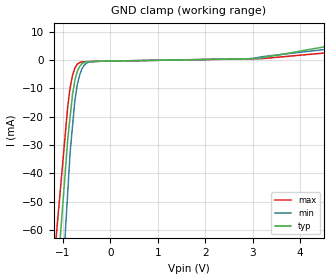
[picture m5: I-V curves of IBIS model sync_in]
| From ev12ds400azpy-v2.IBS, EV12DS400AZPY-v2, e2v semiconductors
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[Model] sync_in
Model_type Input
Vinl = 1.15000V
Vinh = 1.35000V
C_comp 573.000fF 559.000fF 587.000fF
| variable typ   min   max
[Voltage Range] 3.30000V 3.15000V 3.45000V
[POWER Clamp Reference] 3.30000V 3.15000V 3.45000V
[GND Clamp Reference] 0.00000V 0.00000V 0.00000V
[Temperature Range]   25   110   -40
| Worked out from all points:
|   GND clamp passes 1 mA (typ) near -0.57 V on its own axis
[GND Clamp]
-3.3V     -556.2mA   -716.5mA   -469.2mA
-900mV    -27.91mA   -46.58mA   -16.34mA
-850mV    -20.04mA   -32.62mA   -9.785mA
-800mV    -12.18mA   -23.45mA   -5.383mA
-750mV    -7.147mA   -14.29mA   -2.781mA
-700mV    -3.992mA   -8.686mA   -1.463mA
-650mV    -2.306mA   -5.331mA   -888.1uA
-600mV    -1.286mA   -3.039mA   -609.2uA
-550mV    -785.3uA   -1.74mA    -578.7uA
-450mV    -530.2uA   -687uA     -517.8uA
3.15V     668uA      1.043mA    518uA
6.6V      10.84mA    7.725mA    5.659mA
[POWER Clamp]
-3.3V     0A         0A         0A
-350mV    0A         0A         0A
-250mV    0A         0A         0A
-125mV    0A         0A         0A
6.6V      0A         0A         0A
